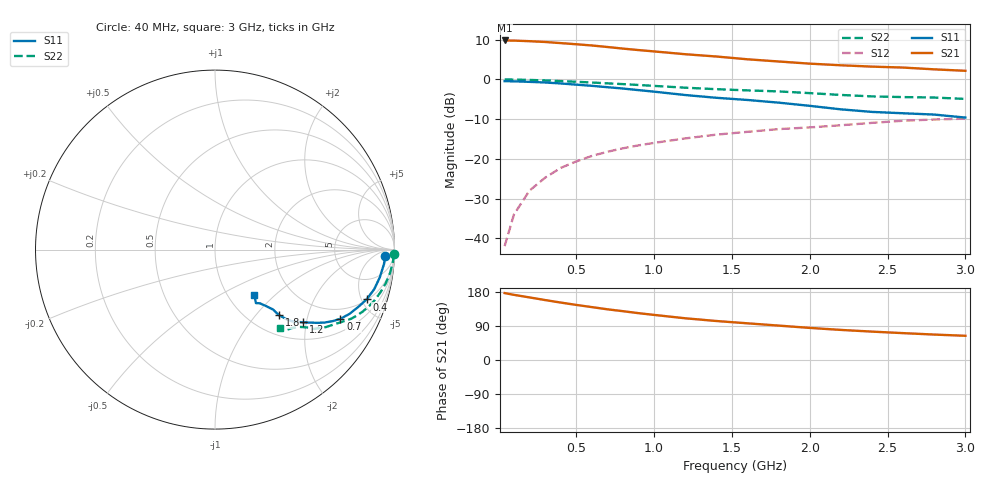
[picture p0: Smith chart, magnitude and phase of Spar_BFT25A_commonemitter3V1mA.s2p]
! Filename:  BFT25AI.S2P  Version:  2.0
! NXP part #: BFT25A  Date: Aug 1990
! Bias condition: Vce=3V, Ic=1mA
#  MHz  S  MA  R  50
! Freq  S11  S21  S12  S22  !GUM [dB]
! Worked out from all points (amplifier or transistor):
!   21 points, 40 MHz to 3 GHz, reference 50 ohm
!   highest |S21| = 9.8 dB at 40 MHz (marker M1)
!   |S21| within 3 dB of that: start of sweep to 1.069 GHz
!   unconditionally stable (mu >= 1): 2.211 GHz to end of sweep
!   at 300 MHz: K = 0.21, MSG = 17.1 dB, |S12| = -24.7 dB
!   at 1 GHz: K = 0.60, MSG = 11.5 dB, |S12| = -16.0 dB
!   at 3 GHz: K = 1.09, MAG = 4.2 dB, |S12| = -9.9 dB
!   S11 on the Smith chart (normalised r, x): 40 MHz: 26, -18; 400 MHz: 2.07, -5.48; 700 MHz: 1.52, -3.22; 1.2 GHz: 1.40, -1.91; 1.8 GHz: 1.35, -1.33; 3 GHz: 1.31, -0.74
40  0.95 -2.1  3.086 176.6  0.008 83.9  0.997 -1.5
100  0.945 -4.9  3.073 171.9  0.02 85.2  0.994 -3.8
200  0.931 -9.6  3.021 165.1  0.04 83.4  0.984 -7.6
300  0.914 -14.0  2.953 158.2  0.058 80.5  0.97 -11.1
400  0.889 -18.2  2.858 151.6  0.077 77.5  0.952 -14.5
500  0.859 -21.9  2.766 145.4  0.093 75.4  0.933 -17.6
600  0.83 -25.6  2.669 139.6  0.109 73.4  0.913 -20.4
700  0.798 -28.9  2.554 133.8  0.123 71.5  0.892 -22.8
800  0.767 -31.3  2.438 128.8  0.136 69.5  0.872 -24.9
900  0.733 -33.7  2.336 123.6  0.148 68.1  0.851 -26.9
1000  0.701 -35.6  2.247 119.0  0.159 66.8  0.828 -28.6
1200  0.636 -39.6  2.072 110.1  0.181 63.9  0.786 -31.9
1400  0.587 -42.9  1.939 102.9  0.202 62.4  0.753 -35.0
1600  0.551 -44.4  1.789 96.8  0.219 60.8  0.727 -37.0
1800  0.51 -45.7  1.679 90.8  0.237 59.5  0.706 -38.8
2000  0.465 -45.9  1.577 84.7  0.249 57.4  0.672 -40.2
2200  0.42 -48.1  1.505 79.4  0.265 56.0  0.637 -42.5
2400  0.39 -50.1  1.447 74.9  0.284 54.5  0.611 -45.7
2600  0.375 -52.6  1.408 70.9  0.302 53.2  0.599 -48.6
2800  0.361 -51.4  1.337 67.1  0.313 52.6  0.591 -49.7
3000  0.331 -49.3  1.282 63.9  0.321 52.0  0.568 -50.4
